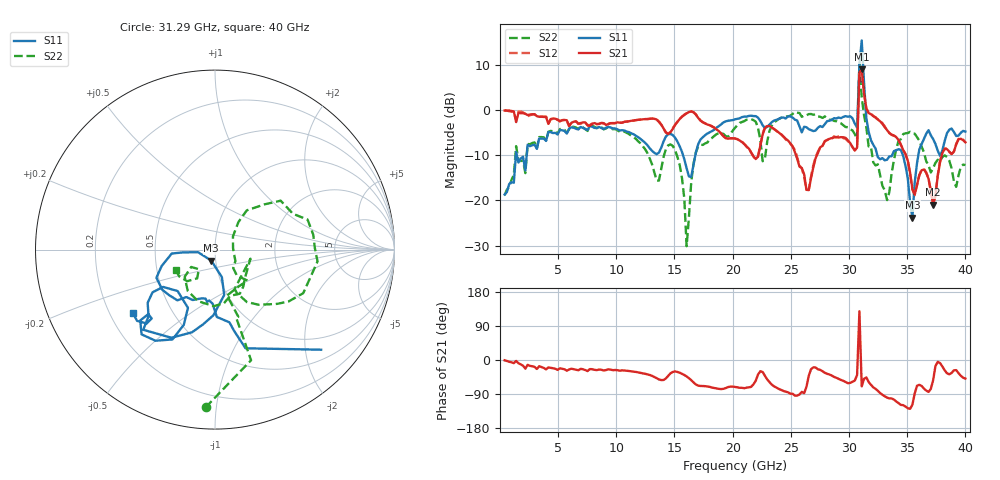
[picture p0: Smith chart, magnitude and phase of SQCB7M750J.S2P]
! Network Analyzer HP8722ES.07.66: Jul 25, 2000 Serial No. US39175408
! 27 Oct 2004  11:32:09
! Frequency  S11  S21  S12  S22
# HZ  S  DB R  50
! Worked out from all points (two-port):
!   201 points, 400 MHz to 40 GHz, reference 50 ohm
!   highest |S21| = 9.01 dB at 31.09 GHz (marker M1); lowest = -20.9 dB at 37.23 GHz (marker M2)
!   |S21| within 3 dB of the highest: 30.86 GHz to 31.2 GHz (338.8 MHz wide, 1.09 % of centre)
!   lowest |S11| = -23.8 dB at 35.45 GHz (marker M3), VSWR 1.14, Z = 47.6 - j5.85 ohm
!   |S11| at or under -10 dB: start of sweep to 1.369 GHz; 32.43 GHz to 33.7 GHz (1.267 GHz wide, 3.83 % of centre); 34.63 GHz to 35.96 GHz (1.325 GHz wide, 3.76 % of centre)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
!   |S22| runs from -30.1 to 10.2 dB; largest |S21 - S12| = 0.32
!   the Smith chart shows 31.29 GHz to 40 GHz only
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4e8  -18.70 -95.1  -0.10 -0.8  -0.03 -0.1  -18.84 -92.3
1.39e9  -9.28 -70.2  -2.66 -2.4  -2.19 -3.2  -7.99 -63.4
7.132e9  -3.94 -103.2  -2.73 -24.3  -2.84 -25.3  -3.84 -123.8
1.3666e10  -9.38 -51.0  -2.60 -51.3  -2.56 -51.2  -15.62 -82.7
1.5052e10  -6.14 -57.5  -3.29 -30.2  -3.25 -30.9  -8.83 -107.0
1.6042e10  -12.86 -48.5  -0.71 -43.4  -0.69 -43.8  -30.12 -173.3
1.7032e10  -7.59 20.8  -1.70 -67.6  -1.70 -68.0  -8.07 1.2
2.02e10  -2.05 16.7  -6.29 -71.1  -6.29 -70.9  -3.93 -10.7
2.2576e10  -3.37 1.1  -5.42 -31.7  -5.19 -32.3  -11.32 -36.6
2.515e10  -1.65 -12.1  -8.01 -89.0  -8.07 -94.3  -0.86 -11.0
2.6932e10  -4.65 -150.9  -12.65 -19.3  -12.21 -19.8  -1.03 -22.6
2.8714e10  -1.78 114.7  -6.06 -44.6  -5.80 -47.0  -2.40 -34.6
3.0694e10  -3.86 57.0  -8.31 -39.4  -8.11 -39.4  -6.48 -75.3
3.0892e10  10.03 -25.2  8.33 128.5  9.09 123.9  10.24 -38.3
3.109e10  15.41 -20.5  9.01 -69.6  8.87 -70.3  2.83 -149.8
3.1288e10  6.11 -45.4  3.76 -49.8  3.77 -49.8  -1.10 -93.4
3.1486e10  -1.80 -43.3  0.36 -45.9  0.34 -47.1  -3.76 -71.9
3.3466e10  -10.25 -113.8  -5.07 -101.3  -5.09 -102.3  -18.12 36.3
3.5446e10  -23.78 -108.9  -17.45 -118.0  -17.61 -118.7  -5.11 -15.2
3.604e10  -8.73 -91.4  -14.41 -65.4  -14.36 -64.9  -6.75 -41.2
3.7228e10  -6.41 -141.7  -20.94 -53.4  -20.82 -51.3  -12.82 -42.7
4e10  -4.77 -142.4  -7.13 -49.0  -7.13 -49.1  -12.15 -152.6
